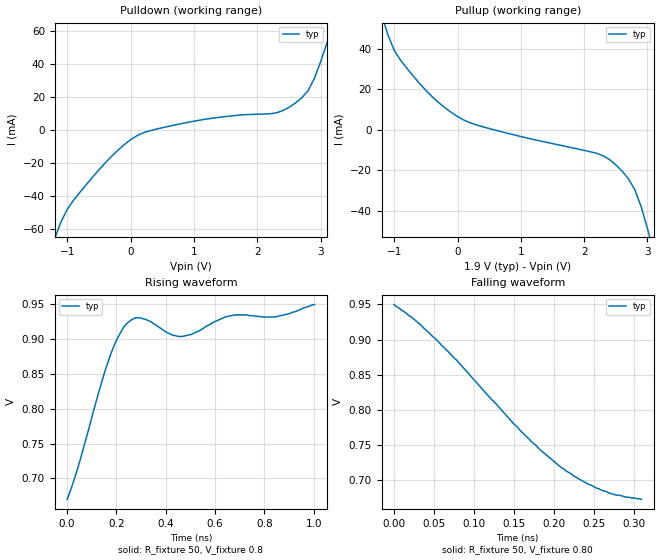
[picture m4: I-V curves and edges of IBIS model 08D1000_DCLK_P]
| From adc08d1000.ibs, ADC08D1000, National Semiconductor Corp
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[Model]   08D1000_DCLK_P
Model_type Output
Polarity Non-Inverting
Vref=0.80
Vmeas=0.80
Rref=50   | 100 Ohms Across Outputs OUTP and OUTM
Cref=5p
|   TYP   MIN   MAX
C_comp   1.5p   1.5p   1.5p
[Temperature Range] 25   85   -40
[Voltage Range]   1.90   1.80   2.00
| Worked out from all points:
|   slope of the pulldown table from 0 to 0.285 V, typ, clamps not added: 55 ohm
|   slope of the pullup table from 0 to 0.285 V, typ, clamps not added: 71.7 ohm
|   falling waveform, R_fixture 50, V_fixture 0.80: 20-80 % time 141ps typ, NA min, NA max; typ from 0.95 V to 0.673 V
|   rising waveform, R_fixture 50, V_fixture 0.8: 20-80 % time 142ps typ, NA min, NA max; typ from 0.67 V to 0.95 V
[Pullup]
|Vtable   I(typ)   I(min)   I(max)
-1.9V     500.5mA    NA         NA
-1.2V     56.89mA    NA         NA
-1.1V     46.81mA    NA         NA
-1V       39.2mA     NA         NA
-700mV    26.55mA    NA         NA
0V        6.503mA    NA         NA
2.3V      -12.88mA   NA         NA
2.7V      -24.28mA   NA         NA
2.8V      -29.62mA   NA         NA
3V        -48.79mA   NA         NA
3.1V      -60.97mA   NA         NA
3.8V      -632.9mA   NA         NA
[Pulldown]
|V(pulldown)   I(typ)   I(min)   I(max)
-1.9V     -639.9mA   NA         NA
-1.2V     -65.95mA   NA         NA
-900mV    -42.64mA   NA         NA
-500mV    -24.26mA   NA         NA
-100mV    -8.986mA   NA         NA
200mV     -1.841mA   NA         NA
2.3V      10.26mA    NA         NA
2.5V      13.57mA    NA         NA
2.8V      23.58mA    NA         NA
2.9V      30.96mA    NA         NA
3.2V      64.9mA     NA         NA
3.8V      501.4mA    NA         NA
[Ramp]
|   TYP   MIN   MAX
dV/dt_r   164mv/.138ns   NA   NA
dV/dt_f   164mv/.142ns   NA   NA
R_load=50
[Falling Waveform]
R_fixture=50
V_fixture=0.80
|Time   V(typ)   V(min)   V(max)
0s        950mV      NA         NA
21.9ps    932mV      NA         NA
53.2ps    900mV      NA         NA
78.2ps    871mV      NA         NA
159.4ps   769mV      NA         NA
209.4ps   718mV      NA         NA
225ps     706mV      NA         NA
259.4ps   686mV      NA         NA
278.2ps   679mV      NA         NA
309.4ps   673mV      NA         NA
[Rising Waveform]
R_fixture=50
V_fixture=0.8
|Time   V(typ)   V(min)   V(max)
0s        670mV      NA         NA
40.6ps    712mV      NA         NA
178.1ps   880mV      NA         NA
228.1ps   917mV      NA         NA
253.1ps   926mV      NA         NA
315.6ps   929mV      NA         NA
465.6ps   904mV      NA         NA
640.6ps   932mV      NA         NA
840.6ps   932mV      NA         NA
1.003ns   950mV      NA         NA
